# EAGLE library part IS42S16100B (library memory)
512K Words x 16 Bits x 2 Banks (16-MBIT) SYNCHRONOUS DYNAMIC RAM Source: www.issi.com .. IS42S16100.pdf
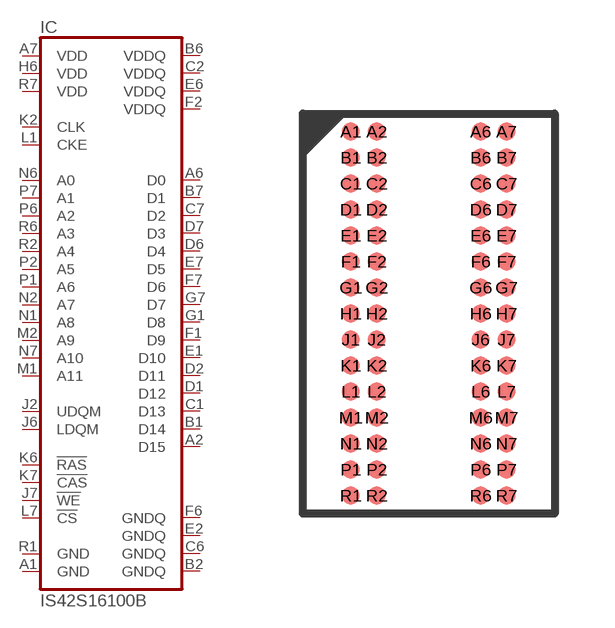
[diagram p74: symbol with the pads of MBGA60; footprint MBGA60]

Designator prefix IC

## IS42S16100B  [MBGA60]
A1  GND  pwr
A2  D15
A6  D0
A7  VDD  pwr
B1  D14
B2  GNDQ  pwr
B6  VDDQ  pwr
B7  D1
C1  D13
C2  VDDQ  pwr
C6  GNDQ  pwr
C7  D2
D1  D12
D2  D11
D6  D4
D7  D3
E1  D10
E2  GNDQ  pwr
E6  VDDQ  pwr
E7  D5
F1  D9
F2  VDDQ  pwr
F6  GNDQ  pwr
F7  D6
G1  D8
G7  D7
H6  VDD  pwr
J2  UDQM  in
J6  LDQM  in
J7  !WE  in
K2  CLK  in
K6  !RAS  in
K7  !CAS  in
L1  CKE  in
L7  !CS  in
M1  A11  in
M2  A9  in
N1  A8  in
N2  A7  in
N6  A0  in
N7  A10  in
P1  A6  in
P2  A5  in
P6  A2  in
P7  A1  in
R1  GND  pwr
R2  A4  in
R6  A3  in
R7  VDD  pwr

## Footprint MBGA60 (pad centres in mm)
Mimi Ball Grid Array mBGA - 10.1 x 6.4 mm Package Code: B (60 Ball) Source: www.issi.com .. IS42S16100.pdf
smd 0.45 x 0.45: A1 -1.95,4.55; A2 -1.3,4.55; A6 1.3,4.55; A7 1.95,4.55; B1 -1.95,3.9; B2 -1.3,3.9; B6 1.3,3.9; B7 1.95,3.9; C1 -1.95,3.25; C2 -1.3,3.25; C6 1.3,3.25; C7 1.95,3.25; D1 -1.95,2.6; D2 -1.3,2.6; D6 1.3,2.6; D7 1.95,2.6; E1 -1.95,1.95; E2 -1.3,1.95; E6 1.3,1.95; E7 1.95,1.95; F1 -1.95,1.3; F2 -1.3,1.3; F6 1.3,1.3; F7 1.95,1.3; G1 -1.95,0.65; G2 -1.3,0.65; G6 1.3,0.65; G7 1.95,0.65; H1 -1.95,0; H2 -1.3,0; H6 1.3,0; H7 1.95,0; J1 -1.95,-0.65; J2 -1.3,-0.65; J6 1.3,-0.65; J7 1.95,-0.65; K1 -1.95,-1.3; K2 -1.3,-1.3; K6 1.3,-1.3; K7 1.95,-1.3; L1 -1.95,-1.95; L2 -1.3,-1.95; L6 1.3,-1.95; L7 1.95,-1.95; M1 -1.95,-2.6; M2 -1.3,-2.6; M6 1.3,-2.6; M7 1.95,-2.6; N1 -1.95,-3.25; N2 -1.3,-3.25; N6 1.3,-3.25; N7 1.95,-3.25; P1 -1.95,-3.9; P2 -1.3,-3.9; P6 1.3,-3.9; P7 1.95,-3.9; R1 -1.95,-4.55; R2 -1.3,-4.55; R6 1.3,-4.55; R7 1.95,-4.55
